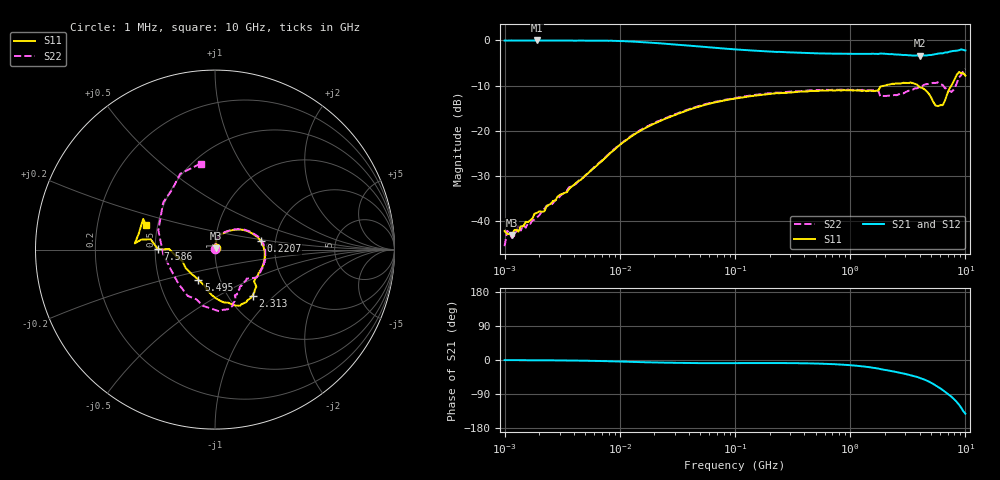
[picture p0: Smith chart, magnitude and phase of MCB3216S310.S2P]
!Agilent Technologies,E5071C,MY46111244,A.11.31
!Date: Thu May 16 16:28:23 2019
!Data & Calibration Information:
!Freq	S11:SOLT2(ON)	S21:SOLT2(ON)	S12:SOLT2(ON)	S22:SOLT2(ON)
# Hz S dB R 50
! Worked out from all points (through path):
!   201 points, 1 MHz to 10 GHz, reference 50 ohm
!   highest |S21| = 0.00 dB at 1.905 MHz (marker M1); lowest = -3.4 dB at 4.008 GHz (marker M2)
!   group delay of S21, straight-line fit = 34.1 ps
!   lowest |S11| = -43.0 dB at 1.159 MHz (marker M3), VSWR 1.01, Z = 50.3 + j0.631 ohm
!   |S11| at or under -10 dB: start of sweep to 1.975 GHz; 3.892 GHz to 7.554 GHz (3.661 GHz wide, 64 % of centre)
!   |S22| runs from -45.5 to -6.3 dB; largest |S21 - S12| = 0.022
!   S11 on the Smith chart (normalised r, x): 1 MHz: 1.01, +0.01; 220.7 MHz: 1.67, +0.17; 2.313 GHz: 1.29, -0.74; 5.495 GHz: 0.79, -0.27; 7.586 GHz: 0.52, +0.00; 10 GHz: 0.43, +0.14
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1000000  -42.13 66.5  -0.02 -0.3  0.11 -0.4  -45.47 68.1
1053043  -42.77 63.7  -0.04 -0.3  0.15 -0.4  -42.09 68.9
1159128  -42.97 62.0  -0.01 -0.5  0.10 -0.5  -43.61 70.8
1318257  -42.26 72.2  -0.02 -0.5  0.13 -0.5  -40.76 68.6
1380384  -41.06 70.8  -0.01 -0.5  0.13 -0.6  -42.02 78.1
1905461  -38.11 77.1  -0.00 -0.7  0.13 -0.8  -39.16 73.2
4810209  -30.33 82.0  -0.04 -1.9  0.13 -1.9  -30.31 83.9
1.106086e7  -22.25 73.2  -0.17 -4.5  -0.02 -4.5  -22.10 73.5
2.206931e7  -17.87 53.7  -0.62 -6.7  -0.48 -6.8  -17.74 53.9
1.047129e8  -12.77 21.8  -2.01 -8.2  -1.86 -8.2  -12.63 22.2
2.206931e8  -11.71 10.6  -2.51 -8.0  -2.36 -8.0  -11.56 11.1
4.810209e8  -11.15 -2.0  -2.83 -9.1  -2.68 -9.2  -11.03 -0.6
1.269299e9  -11.18 -25.3  -2.97 -16.6  -2.78 -16.6  -10.91 -21.3
2.206931e9  -9.72 -49.1  -3.04 -28.3  -2.87 -28.3  -12.17 -50.9
2.312765e9  -9.58 -50.5  -3.01 -29.5  -2.89 -29.5  -12.20 -52.6
4.008491e9  -10.32 -76.1  -3.39 -47.2  -3.20 -47.2  -10.25 -69.1
5.495409e9  -14.38 -118.9  -3.04 -66.8  -2.88 -66.8  -9.41 -82.7
6.369884e9  -14.30 -160.3  -2.84 -79.6  -2.63 -79.5  -9.88 -102.0
7.585776e9  -9.93 179.4  -2.38 -97.1  -2.23 -97.1  -11.38 -155.0
8.792888e9  -6.97 175.5  -2.17 -117.7  -2.01 -117.7  -8.18 137.8
9.597629e9  -7.23 156.9  -2.09 -135.2  -1.91 -135.3  -6.65 114.7
1e10  -7.78 160.0  -2.21 -141.8  -2.03 -141.7  -6.27 99.5
